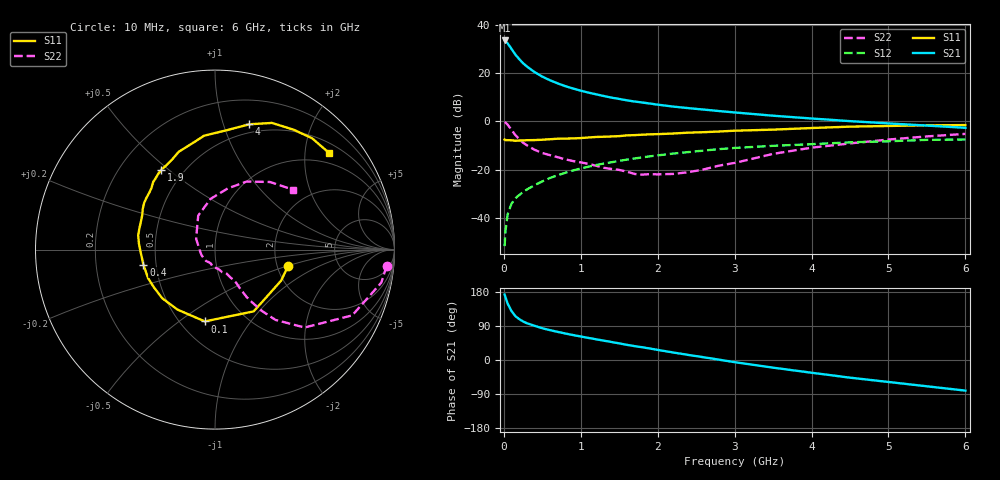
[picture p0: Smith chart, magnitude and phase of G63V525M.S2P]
! SIEMENS Small Signal Semiconductors
! BFG193
! Si NPN RF Bipolar Junction Transistor in SOT223
! VCE = 3.5 V  IC = 25 mA
! Common Emitter S-Parameters:  August  1996
# GHz  S  MA  R  50
!  f  S11  S21  S12  S22
! GHz  MAG  ANG  MAG  ANG  MAG  ANG  MAG  ANG
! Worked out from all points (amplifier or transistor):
!   36 points, 10 MHz to 6 GHz, reference 50 ohm
!   highest |S21| = 33.4 dB at 10 MHz (marker M1)
!   |S21| within 3 dB of that: start of sweep to 88.94 MHz
!   unconditionally stable (mu >= 1): 648.3 MHz to 2.434 GHz
!   at 250 MHz: K = 0.80, MSG = 26.7 dB, |S12| = -29.3 dB
!   at 1.4 GHz: K = 1.05, MAG = 12.0 dB, |S12| = -17.0 dB
!   at 6 GHz: K = 0.89, MSG = 2.4 dB, |S12| = -7.6 dB
!   S11 on the Smith chart (normalised r, x): 10 MHz: 2.30, -0.51; 100 MHz: 0.66, -0.63; 400 MHz: 0.42, -0.08; 1.9 GHz: 0.38, +0.47; 4 GHz: 0.42, +1.22; 6 GHz: 0.72, +2.55
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0.01  0.4177 -12.7  46.98 172.7  0.0026 88.1  0.9604 -5.5
0.02  0.4069 -25.2  45.93 166.7  0.0052 83.5  0.9449 -11.2
0.05  0.4061 -57.9  40.89 148.5  0.0119 70.7  0.848 -25.6
0.1  0.4041 -98.1  31.36 129.1  0.0198 63.7  0.6617 -41.0
0.15  0.3942 -122.0  23.98 115.7  0.0255 60.9  0.5168 -49.3
0.2  0.3999 -137.3  19.28 107.9  0.0297 61.0  0.4272 -52.7
0.25  0.4001 -148.5  15.91 101.7  0.0344 61.3  0.3587 -54.9
0.3  0.4054 -156.8  13.55 97.0  0.0387 62.0  0.3179 -56.3
0.4  0.4077 -168.2  10.39 90.2  0.0477 62.5  0.2568 -57.2
0.5  0.4145 -178.0  8.378 83.8  0.0569 63.1  0.2202 -57.5
0.6  0.4245 175.8  7.053 78.8  0.0671 62.7  0.1986 -58.7
0.7  0.4352 169.6  6.079 74.2  0.0762 62.2  0.1803 -60.7
0.9  0.4415 159.1  4.753 65.8  0.096 59.4  0.15 -63.9
1.1  0.4616 150.8  3.913 58.3  0.1146 56.5  0.1312 -72.6
1.4  0.4845 139.1  3.081 47.5  0.1418 50.8  0.1027 -87.2
1.9  0.5364 123.8  2.324 30.2  0.1879 40.7  0.0805 -128.3
2.2  0.5575 115.1  2.012 19.9  0.2142 33.8  0.0813 -158.0
3.5  0.6708 83.8  1.302 -20.2  0.3102 3.3  0.2113 116.3
4  0.7239 74.7  1.14 -33.6  0.3351 -6.4  0.2839 94.9
4.5  0.7738 65.8  1.006 -46.6  0.3663 -16.5  0.3478 78.3
5.5  0.823 48.9  0.814 -69.4  0.4123 -39.8  0.4859 50.8
6  0.8332 40.3  0.732 -80.8  0.4184 -53.3  0.5476 37.6
